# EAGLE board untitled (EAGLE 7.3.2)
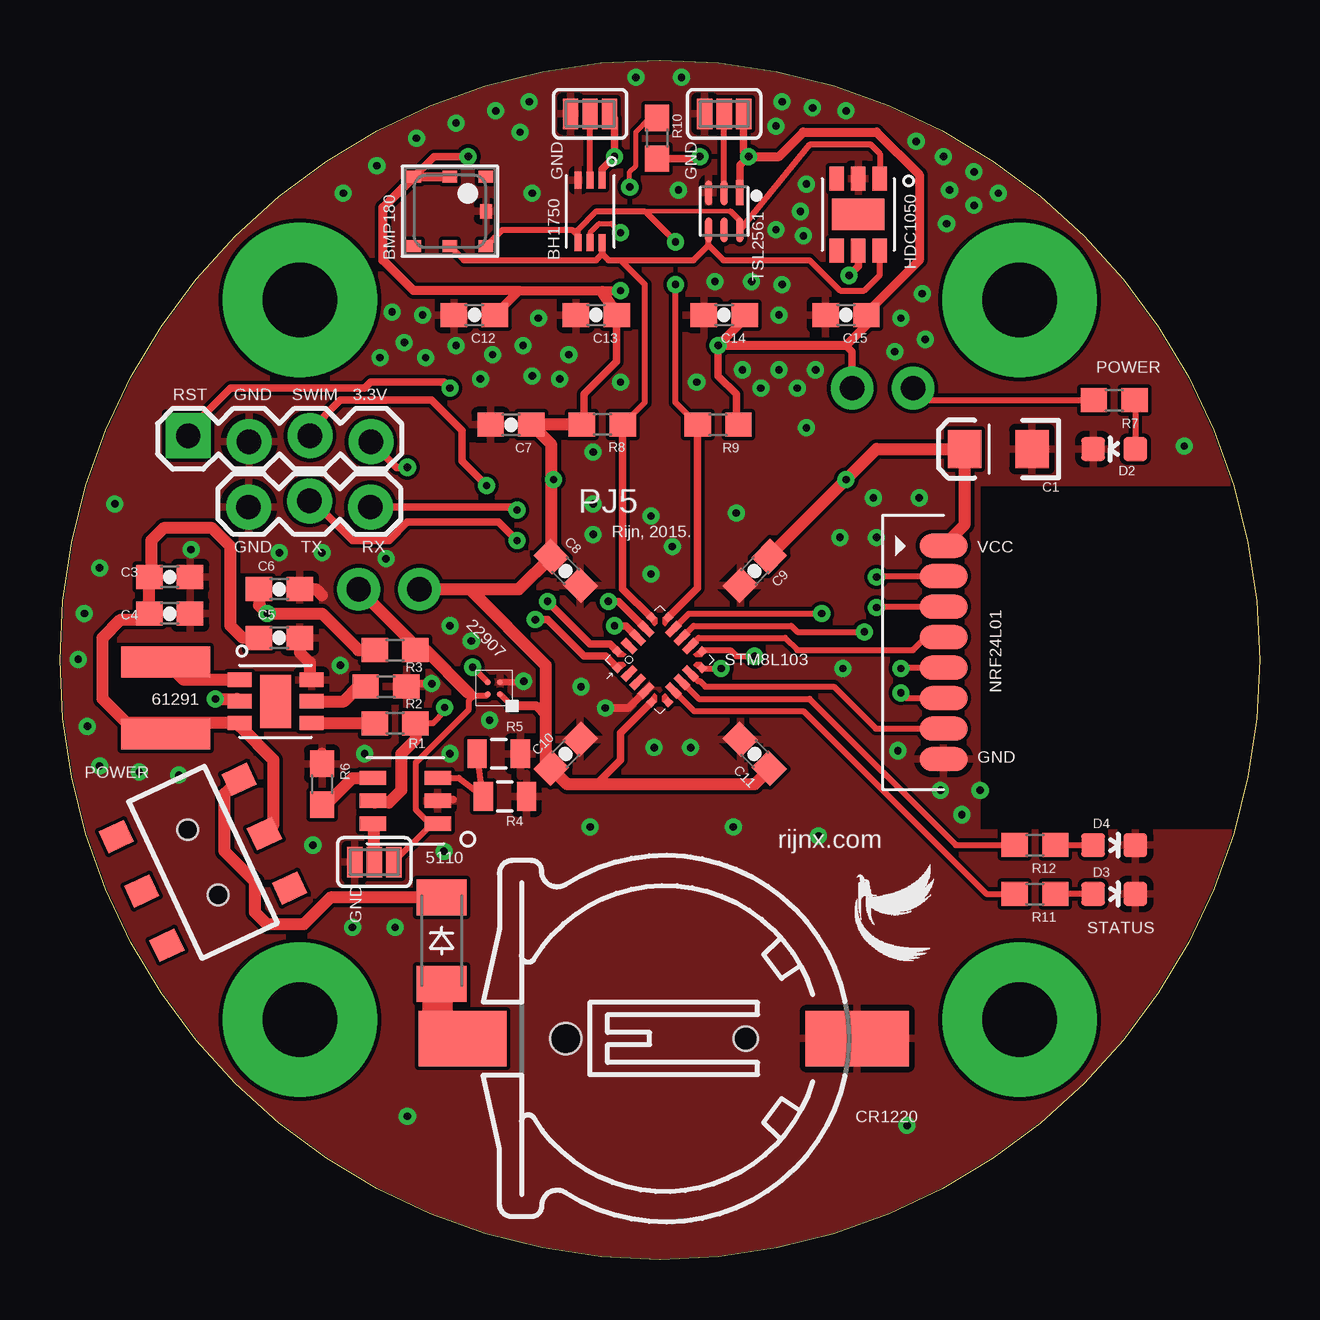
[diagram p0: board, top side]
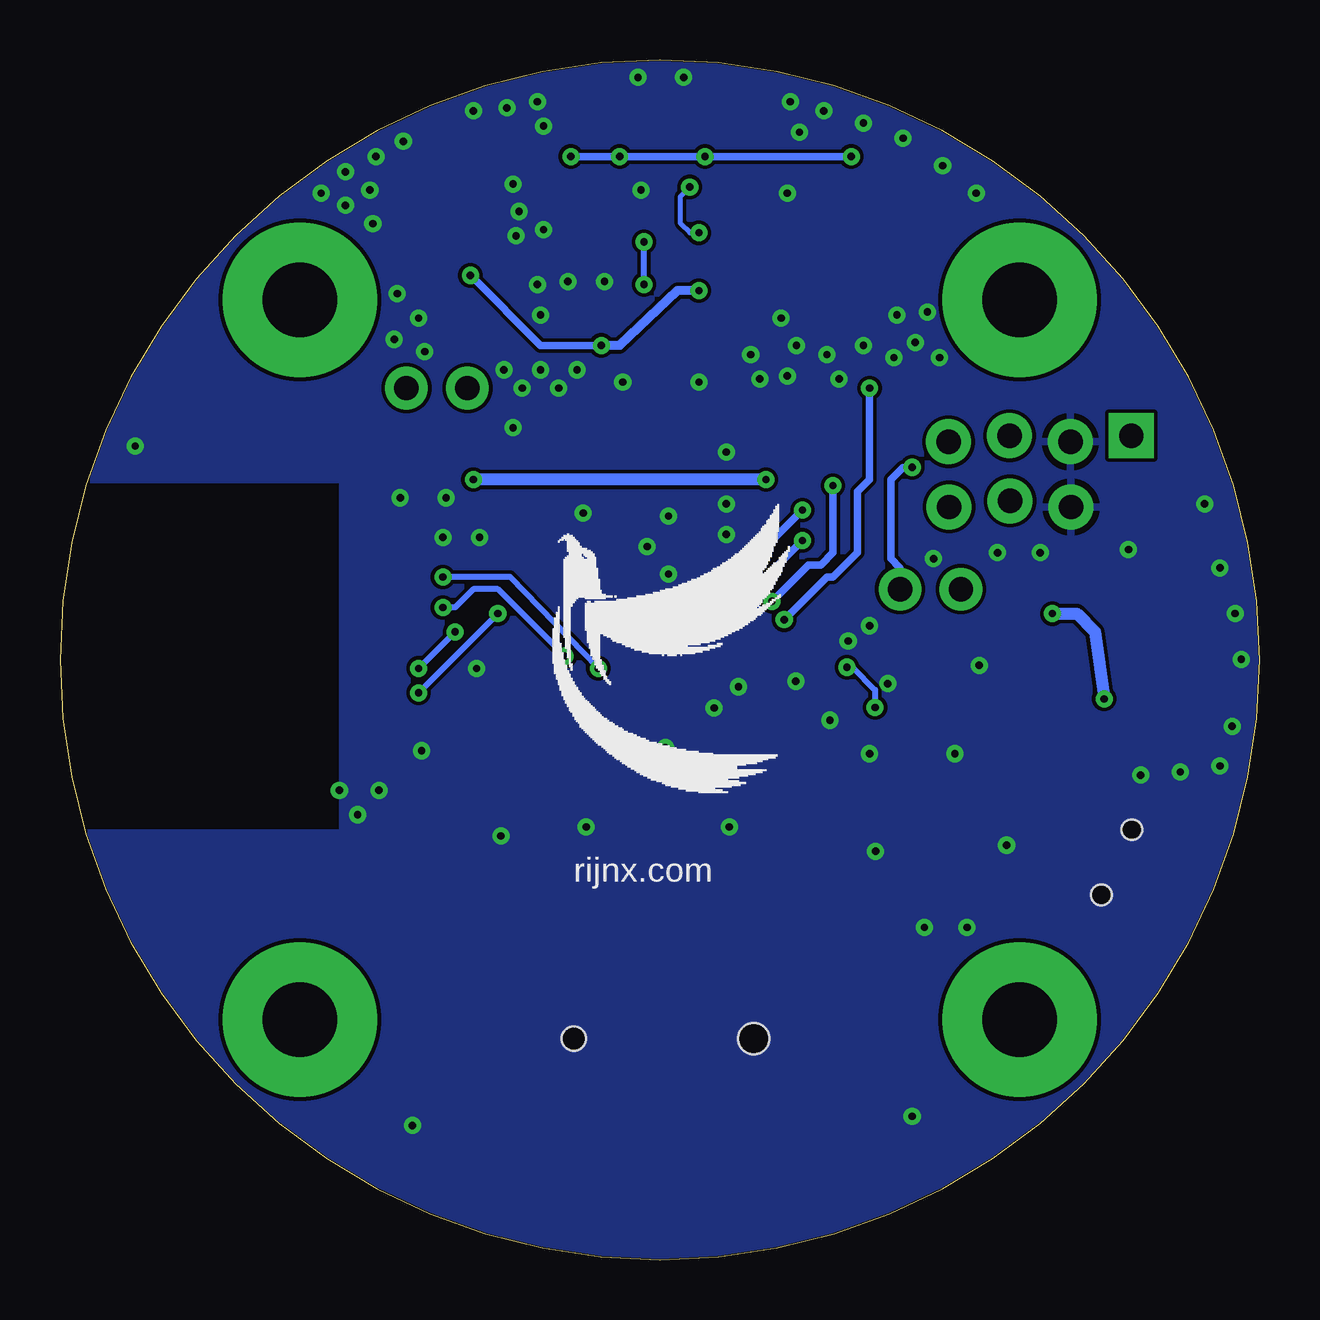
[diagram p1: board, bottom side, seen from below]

Size 50 x 50 mm. Coordinates in mm from the lower left corner, seen from the top.
Outline: 25,50 arc-180 25,0 arc-180 25,50
Copper layers (1*16): Top 0.035mm / dielectric 1.5mm / Bottom 0.035mm
Design rules "default *": minimum track width 6mil, minimum drill 12mil, track to track 6mil, track to pad 6mil, pad to pad 6mil, via to via 6mil, smd to smd 6mil, copper to edge 2mil, drill to drill 6mil, minimum pad ring 10mil, minimum via ring 8mil, stop-mask expansion 4mil, vias tented up to drill 15mil, thermal gap 10mil

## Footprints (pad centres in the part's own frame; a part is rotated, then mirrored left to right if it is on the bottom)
EIA3216 = smd 1.4 x 1.6: A 1.4,0; C -1.4,0
0603-CAP = smd 1.1 x 1: 1 -0.85,0; 2 0.85,0
SOD-123_MINI-SMA = smd 1.5 x 2.1: A 1.8,0; C -1.8,0
LED-0603 = smd 1 x 1: A 0,-0.877; C 0,0.877
CH291-1220LF = smd 2.3 x 3.66: + 0,-2.296 | smd 2.3 x 4.3: - 0,14.146 | hole 1.3: 0,2 | hole 1: 0,9.5
1X03_LOCK = drill 1.016 pad 1.88: 1 0,0.127; 2 2.54,-0.127; 3 5.08,0.127
1X04_LOCK = drill 1.016 pad 1.88 square: 1 0,0.127 | drill 1.016 pad 1.88: 2 2.54,-0.127; 3 5.08,0.127; 4 7.62,-0.127
0603 = smd 1.1 x 1: 1 -0.85,0; 2 0.85,0
0805 = smd 0.8 x 1.2: 1 -0.9,0; 2 0.9,0
AYZ0202 = smd 1 x 1.15: 1 -2.5,2.825; 2 0,2.825; 3 2.5,2.825; 4 -2.5,-2.825; 5 0,-2.825; 6 2.5,-2.825 | hole 0.85: 1.5,0; -1.5,0
PAD-JUMPER-3-NC_BY_PASTE_YES_SILK_FULL_BOX = smd 0.635 x 1.27: 1 -0.813,0; 2 0,0; 3 0.813,0
PTH-JUMPER-2-NO_NO_SILK = drill 1.016 pad 1.778: 1 -1.27,0; 2 1.27,0
BMP180 = smd 0.6 x 0.5: 1 1.5,1.45; 2 0,1.45; 3 -1.5,1.45; 4 -1.5,-1.45; 5 0,-1.45; 6 1.5,-1.45 | smd 0.5 x 0.6: 7 1.5,0
FN-6 = smd 1.05 x 0.3: 1 -0.775,0.65; 2 -0.775,0; 3 -0.775,-0.65; 4 0.775,-0.65; 5 0.775,0; 6 0.775,0.65
SWPA4018S = smd 1.3 x 3.7: P$1 -1.5,0; P$2 1.5,0
PWSON-N6 = smd 0.6 x 1: P$1 0.9,1.5; P$2 0,1.5; P$3 -0.9,1.5; P$4 -0.9,-1.5; P$5 0,-1.5; P$6 0.9,-1.5 | smd 2.2 x 1.3: P$7 0,0
DDC(R-PDSO-G6) = smd 0.6 x 1.1: P$1 -0.95,-1.35; P$2 0,-1.35; P$3 0.95,-1.35; P$4 0.95,1.35; P$5 0,1.35; P$6 -0.95,1.35
YZT(S-XBGA-N4) = smd 0.25 x 0.25: P$A1 0.25,-0.25; P$A2 -0.25,-0.25; P$B1 0.25,0.25; P$B2 -0.25,0.25
UFQFPN20 = smd 0.3 x 0.3: P$1 -1.5,1; P$5 -1.5,-1; P$6 -1,-1.5; P$10 1,-1.5; P$11 1.5,-1; P$15 1.5,1; P$16 1,1.5; P$20 -1,1.5 | smd 0.7 x 0.3: P$2 -1.3,0.5; P$3 -1.3,0; P$4 -1.3,-0.5; P$12 1.3,-0.5; P$13 1.3,0; P$14 1.3,0.5 | smd 0.3 x 0.7: P$7 -0.5,-1.3; P$8 0,-1.3; P$9 0.5,-1.3; P$17 0.5,1.3; P$18 0,1.3; P$19 -0.5,1.3
M08-1.27 = smd 1 x 2: P$1 0,0; P$2 1.27,0; P$3 2.54,0; P$4 3.81,0; P$5 5.08,0; P$6 6.35,0; P$7 7.62,0; P$8 8.89,0
WSOF-6 = smd 0.3 x 0.7: P$1 -0.5,-1.3; P$2 0,-1.3; P$3 0.5,-1.3; P$4 0.5,1.3; P$5 0,1.3; P$6 -0.5,1.3

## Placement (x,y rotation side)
C1  10uF  [EIA3216]  39.12,33.78 180 top
C3  100pF  [0603-CAP]  4.57,28.45 0 top
C4  0.1uF  [0603-CAP]  4.57,26.92 0 top
C5  10uF  [0603-CAP]  9.14,25.91 0 top
C6  22uF  [0603-CAP]  9.14,27.94 0 top
C7  1.0uF  [0603-CAP]  18.8,34.8 180 top
C8  0.1uF  [0603-CAP]  21.08,28.7 315 top
C9  0.1uF  [0603-CAP]  28.96,28.7 225 top
C10  0.1uF  [0603-CAP]  21.08,21.08 45 top
C11  0.1uF  [0603-CAP]  28.96,21.08 135 top
C12  0.1uF  [0603-CAP]  17.27,39.37 180 top
C13  0.1uF  [0603-CAP]  22.35,39.37 180 top
C14  0.1uF  [0603-CAP]  27.69,39.37 180 top
C15  0.1uF  [0603-CAP]  32.77,39.37 180 top
D1  B0520LW  [SOD-123_MINI-SMA]  15.91,13.29 270 top
D2  Yellow  [LED-0603]  43.94,33.78 90 top
D3  Yellow  [LED-0603]  43.94,15.24 270 top
D4  Yellow  [LED-0603]  43.94,17.27 270 top
G1  CH291-1220LF  [CH291-1220LF]  19.08,9.21 270 top
JP1  [1X03_LOCK]  12.94,31.49 180 top
JP2  [1X04_LOCK]  5.34,34.21 0 top
R1  0  [0603]  13.97,22.35 180 top
R2  0  [0603]  13.59,23.88 180 top
R3  0  [0603]  13.97,25.4 180 top
R4  40.2K  [0805]  18.54,19.3 180 top
R5  48.7K  [0805]  18.29,21.08 180 top
R6  10K  [0603]  10.92,19.81 270 top
R7  500  [0603]  43.94,35.81 180 top
R8  4.7K  [0603]  22.61,34.8 0 top
R9  4.7K  [0603]  27.43,34.8 180 top
R10  1K  [0603]  24.89,46.74 270 top
R11  500  [0603]  40.64,15.24 180 top
R12  500  [0603]  40.64,17.27 180 top
S1  AYZ0202  [AYZ0202]  5.96,16.56 295 top
SJ1  JUMPER-PAD-3-NC_BY_PASTE  [PAD-JUMPER-3-NC_BY_PASTE_YES_SILK_FULL_BOX]  13.1,16.57 180 top
SJ2  JUMPER-BYPASS  [PTH-JUMPER-2-NO_NO_SILK]  13.72,27.94 180 top
SJ3  JUMPER-POWERLED  [PTH-JUMPER-2-NO_NO_SILK]  34.29,36.32 180 top
SJ4  JUMPER-PAD-3-NC_BY_PASTE  [PAD-JUMPER-3-NC_BY_PASTE_YES_SILK_FULL_BOX]  27.69,47.75 180 top
SJ5  JUMPER-PAD-3-NC_BY_PASTE  [PAD-JUMPER-3-NC_BY_PASTE_YES_SILK_FULL_BOX]  22.1,47.75 0 top
U1  BMP180  [BMP180]  16.26,43.69 0 top
U2  TSL2561FN  [FN-6]  27.69,43.69 270 top
U$1  SWPA4018S3R3MT  [SWPA4018S]  4.41,23.41 90 top
U$2  TPS61291  [PWSON-N6]  8.98,23.27 90 top
U$3  TPL5110  [DDC(R-PDSO-G6)]  14.4,19.12 90 top
U$4  TPS22907  [YZT(S-XBGA-N4)]  18.09,23.81 0 top
U$5  STM8L101  [UFQFPN20]  25,25 45 top
U$6  NRF24L01_MODULE_SMD  [M08-1.27]  36.83,29.75 270 top
U$7  HDC1050  [PWSON-N6]  33.27,43.56 0 top
U$8  BH1750  [WSOF-6]  22.1,43.69 180 top
U$9  [LOGO-3]  29.51,19.41 0 bottom
U$10  [LOGO-1]  33.12,12.43 0 top

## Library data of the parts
C1 = SparkFun-Capacitors; PROD_ID: CAP-00811
C3-C6 = SparkFun-Capacitors; PROD_ID: CAP-07883
C7 = SparkFun-Capacitors; PROD_ID: CAP-00868
C8-C15 = SparkFun-Capacitors; PROD_ID: CAP-08604
D1 = diode
D2-D4 = SparkFun-LED; PROD_ID: DIO-09003
G1 = battery
JP1 JP2 = SparkFun-Connectors
R1-R3 R6-R12 = SparkFun-Resistors; PROD_ID: RES-08306
R4 R5 = SparkFun-Resistors; PROD_ID: RES-09883
S1 = SparkFun-Electromechanical; PROD_ID: SWCH-08179; SF_ID: COM-00597
SJ1-SJ5 = SparkFun-Passives
U1 U2 = SparkFun-Sensors
U$1-U$4 U$6-U$10 = User-Submitted
U$5 = st-microelectronics; DEVICE: STM8F101

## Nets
3.3V: R3.1 SJ1.1 SJ2.2 U$3.P$1 U$4.P$A2
DONE: R6.2 U$3.P$4
GND: C1.C C3.2 C4.2 C5.2 C6.2 C7.2 C8.2 C9.2 C10.2 C11.2 C12.2 C13.2 C14.2 C15.2 D2.C D3.C D4.C G1.- JP1.3 JP2.2 R2.1 R4.1 R5.1 R6.1 SJ1.3 SJ4.3 SJ5.1 U1.7 U2.3 U$2.P$6 U$3.P$2 U$4.P$B1 U$5.P$4 U$6.P$8 U$7.P$2 U$8.P$3
I2C_INT: U2.5
I2C_SCL: R8.2 U1.5 U2.4 U$5.P$16 U$7.P$6 U$8.P$6
I2C_SDA: R9.2 U1.6 U2.6 U$5.P$15 U$7.P$1 U$8.P$4
MESH: C1.A C7.1 C8.1 C9.1 C10.1 C11.1 C12.1 C13.1 C14.1 C15.1 JP2.4 R8.1 R9.1 R10.2 SJ2.1 SJ3.2 SJ4.1 SJ5.3 U1.2 U1.3 U2.1 U$4.P$A1 U$5.P$5 U$6.P$1 U$7.P$5 U$8.P$1
N$1: D1.A G1.+
N$2: D1.C S1.1
N$3: U$1.P$2 U$2.P$1
N$4: C6.1 R3.2 U$2.P$2
N$5: R1.2 U$2.P$4
N$6: R2.2 U$2.P$5
N$7: R4.2 R5.2 U$3.P$3
N$8: R7.2 SJ3.1
N$9: D2.A R7.1
N$10: SJ1.2 U$3.P$6
N$11: SJ4.2 U2.2
N$12: SJ5.2 U$8.P$2
N$13: R10.1 U$8.P$5
N$14: D3.A R11.1
N$15: D4.A R12.1
N$16: R11.2 U$5.P$7
N$17: R12.2 U$5.P$8
NRF_CE: U$5.P$10 U$6.P$2
NRF_CSN: U$5.P$11 U$6.P$3
NRF_IRQ: U$5.P$9 U$6.P$7
RST: JP2.1 U$5.P$1
SPI_MISO: U$5.P$14 U$6.P$6
SPI_MOSI: U$5.P$13 U$6.P$5
SPI_SCK: U$5.P$12 U$6.P$4
SWIM: JP2.3 U$5.P$20
TPL_DRV: R1.1 U$3.P$5 U$4.P$B2
UART_RX: JP1.1 U$5.P$17
UART_TX: JP1.2 U$5.P$18
V_BATT: C3.1 C4.1 C5.1 S1.2 U$1.P$1 U$2.P$3

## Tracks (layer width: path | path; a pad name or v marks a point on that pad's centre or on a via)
3.3V
  Top 0.254: 17.02,23.62 17.17,23.62 17.27,23.52 | 17.27,23.52 17.8,23.52 U$4.P$A2 | U$3.P$1 15.4,18.17 | 15.4,18.17 14.83,18.75 14.83,20.73 17.04,22.94 17.04,23.29 17.27,23.52 | 15.4,18.17 15.4,18.06 SJ1.1
  Top 0.508: SJ2.2 14.82,25.57 R3.1 15.24,25.4 17.02,23.62
DONE
  Top 0.508: R6.2 11.09,18.96 12.19,20.07 U$3.P$4
GND  (via drill 0.3)
  Top 0.254: U$4.P$B1 19.29,24.06 v19.33,24.11
  Top 0.305: R2.1 14.95,24 v15.49,24 | U$3.P$2 15.8,19.18 16.38,19.18 | U$5.P$4 23.69,22.99 v22.73,22.99
  Top 0.508: C5.2 9.99,25.31 10.41,24.89 10.41,24.24 U$2.P$6 | C6.2 10.67,27.94 10.92,27.69 | R6.1 10.92,21.08
  other vias: 11.68,24.77 21.21,37.72 19.68,36.83 18.03,37.72 14.35,38.23 11.81,44.45 19.68,44.45 30.1,48.26 30.1,40.64 25.78,44.58 16.26,26.42 17.14,25.78 22.23,31.5 22.23,30.23 22.23,33.66 2.29,31.5 5.46,29.59 17.91,22.48 21.72,23.88 24.77,21.34 26.29,21.34 31.62,17.65 14.48,5.97 35.31,5.59 28.19,31.11 24.64,30.99 25.53,29.72 24.64,28.57 22.1,18.03 28.07,18.03 32.51,30.1 32.64,24.64 34.92,21.21 34.04,30.1 33.91,31.75 35.81,31.75 46.86,33.91 36.7,19.56 38.35,19.56 37.59,18.54 1.65,28.83 1.02,26.92 0.76,25.02 1.14,22.23 1.65,20.57 3.3,20.32 4.95,20.19 10.54,17.27 9.14,29.46 10.92,29.46 13.59,29.21 12.19,13.84 13.97,13.84 16,17.02 16.26,21.08 31.11,34.67 13.21,45.59 14.86,46.74 16.51,47.37 18.16,47.88 19.56,48.26 19.18,46.99 24,49.28 25.91,49.28 31.37,48.01 32.77,47.88 29.84,47.24 35.69,46.61 36.83,45.97 38.1,45.34 39.12,44.45 37.08,44.58 38.1,43.94 36.96,43.18 35.94,40.26 35.05,39.24 36.07,38.35 34.8,37.85 13.84,39.5 15.11,39.37 13.34,37.59 15.24,37.59 16.51,38.1 17.53,36.7 19.94,39.24 19.3,38.1 20.83,36.7 23.37,36.58 26.54,36.58 28.45,37.08 29.21,36.32 29.97,37.08 30.73,36.32 31.5,37.08 30.86,43.69 29.84,42.93 30.99,42.67 27.3,40.77 28.83,40.77 29.97,39.37 12.7,21.08 31.11,44.83
  pour Top: -1.27,51.31 50.8,51.31 50.8,32.38 38.23,32.38 38.23,17.78 50.93,17.78 50.93,-0.64 -1.27,-0.64
  pour Bottom: 0.13,53.72 53.09,53.72 53.09,32.51 38.23,32.51 38.23,17.78 50.93,17.78 50.93,-0.51 -0.38,-0.51 -0.38,53.72
I2C_SCL
  Top 0.254: U1.5 16.84,41.66 22.35,41.66 22.6,41.9 U$8.P$6 22.61,41.91 22.86,41.66 23.37,41.66 | 23.37,41.66 26.42,41.66 27.04,42.28 | 27.04,42.28 U2.4 | 27.04,42.28 27.66,41.66 31.24,41.66 32.51,40.39 33.53,40.39 34.17,41.03 U$7.P$6 | R8.2 24.38,35.73 24.38,40.64 23.37,41.66
  Top 0.305: U$5.P$16 23.46,27.96 R8.2
I2C_SDA  (via drill 0.3)
  Top 0.178: 27.94,43.69 23.75,43.69
  Top 0.254: U1.6 18.44,42.93 21.34,42.93 21.59,42.67 | 21.59,42.67 21.6,42.66 U$8.P$4 21.59,42.67 | 21.59,42.67 21.59,42.93 22.35,43.69 23.75,43.69 24.38,43.69 v25.65,42.42 | 27.94,43.69 28.34,43.29 U2.6 31.27,46.48 33.78,46.48 34.17,46.09 U$7.P$1 | R9.2 25.65,35.73 v25.65,40.64
  Top 0.305: U$5.P$15 26.58,28 R9.2
  Bottom 0.254: v25.65,40.64 v25.65,42.42
MESH  (via drill 0.3)
  Top 0.178: v20.57,32.51 20.48,32.6 20.48,33.53
  Top 0.254: U$4.P$A1 18.82,23.09
  Top 0.305: U$8.P$1 22.6,45.46 v23.11,45.97 23.11,47.55 SJ5.3 | v17.02,45.97 15.59,45.97 U1.3 | U2.1 28.34,45.61 v28.7,45.97 28.5,46.18 SJ4.1 | U$7.P$5 33.27,41.4 v32.89,41.02 | R10.2 26.58,45.89 v26.67,45.97 | C13.1 23.2,37.43 21.84,36.07 21.84,34.89 R8.1 | v27.43,38.1 27.43,36.83 28.19,36.07 28.19,34.89 R9.1 | SJ3.2 33.02,37.85 32.77,38.1 | U$5.P$5 23.37,21.95 23.37,20.83 22.35,19.81 | JP2.4 14.03,33.02 v14.48,33.02
  Top 0.381: 18.82,23.09 19.84,23.09 20.24,22.68 | C12.1 19.14,40.39 | 19.14,40.39 22.61,40.39 | 22.61,40.39 23.2,39.54 C13.1 22.61,40.22 22.61,40.39 | 22.61,40.39 v23.37,40.39 | C14.1 28.54,39.2 v27.43,38.1 32.77,38.1 33.62,38.95 C15.1 | 19.14,40.39 14.73,40.39 13.46,41.66 13.46,43.84 U1.3 U1.2 | v28.7,45.97 29.97,45.97 30.99,46.99 34.04,46.99 35.81,45.21 35.81,41.66 33.53,39.37
  Top 0.508: C9.1 v32.77,32.51 34.04,33.78 C1.A 37.72,30.64 U$6.P$1 | R8.1 C7.1 20.48,33.96 20.48,33.53 C8.1 19.12,27.94 SJ2.1 17.07,27.94 20.24,24.77 20.24,22.68 20.24,20.72 C10.1 21.15,19.81 22.35,19.81 28.96,19.81 29.56,20.41 C11.1
  Bottom 0.305: v17.02,45.97 v23.11,45.97 v26.67,45.97 v28.7,45.97 | v32.89,41.02 29.97,38.1 v27.43,38.1 | v14.48,33.02 14.86,33.02 15.37,32.51 15.37,29.21 14.99,28.83 SJ2.1
  Bottom 0.381: v23.37,40.39 24.26,40.39 26.67,38.1 v27.43,38.1
  Bottom 0.508: v20.57,32.51 v32.77,32.51
N$1
  Top 1.27: D1.A 15.75,11.49 15.75,9.65 16.79,9.65 G1.+
N$2
  Top 0.508: D1.C 11.28,15.09 10.16,13.97 8.64,13.97 8.13,14.48 8.13,15.75 6.86,17.02 6.86,19.41 S1.1
N$3
  Top 0.508: U$2.P$1 5.16,24.17 U$1.P$2
N$4  (via drill 0.3)
  Top 0.508: C6.1 8.29,27.27 v8.64,26.92 10.92,26.92 12.45,25.4 R3.2 | v6.48,23.37 7.38,23.37 U$2.P$2
  Bottom 0.508: v8.64,26.92 7.62,26.92 6.86,26.16 v6.48,23.37
N$5
  Top 0.508: U$2.P$4 13.11,22.37 R1.2
N$6
  Top 0.508: U$2.P$5 11.84,23.27 12.45,23.88 R2.2
N$7
  Top 0.254: U$3.P$3 16.62,20.07 R4.2 R5.2
N$8
  Top 0.254: SJ3.1 36.07,35.81 R7.2
N$9
  Top 0.254: R7.1 44.82,35.79 D2.A
N$10
  Top 0.508: SJ1.2 13.1,18.12 U$3.P$6
N$11
  Top 0.254: U2.2 SJ4.2
N$12
  Top 0.254: U$8.P$2 SJ5.2
N$13  (via drill 0.3)
  Top 0.203: U$8.P$5 22.1,42.8 22.48,43.18 22.99,43.18 v23.37,42.8 | v23.75,44.7 23.75,45.34 24,45.59 24,46.99 24.6,47.59 R10.1
  Bottom 0.203: v23.37,42.8 23.75,42.8 24.13,43.18 24.13,44.32 v23.75,44.7
N$14
  Top 0.254: D3.A R11.1
N$15
  Top 0.254: R12.1 D4.A
N$16
  Top 0.254: U$5.P$7 26.43,22.86 30.99,22.86 38.61,15.24 R11.2
N$17
  Top 0.254: U$5.P$8 26.63,23.37 31.24,23.37 37.34,17.27 R12.2
N$18  (via drill 3.1 pad 6.45)
  other vias: 40,40
N$19  (via drill 3.1 pad 6.45)
  other vias: 40,10
N$20  (via drill 3.1 pad 6.45)
  other vias: 10,10
N$21  (via drill 3.1 pad 6.45)
  other vias: 10,40
NRF_CE  (via drill 0.3)
  Top 0.254: U$5.P$10 26.78,24.64 v27.56,24.64 | v34.04,28.45 34.07,28.48 U$6.P$2
  Bottom 0.254: v27.56,24.64 31.24,28.45 v34.04,28.45
NRF_CSN  (via drill 0.3)
  Top 0.254: U$5.P$11 26.81,25.4 27.94,25.4 28.19,25.15 v28.96,25.15 | v34.04,27.18 34.07,27.21 U$6.P$3
  Bottom 0.254: v28.96,25.15 31.75,27.94 32.77,27.94 33.53,27.18 v34.04,27.18
NRF_IRQ
  Top 0.254: U$5.P$9 26.6,24.11 26.67,24.11 26.9,23.88 32.26,23.88 34,22.13 U$6.P$7
RST  (via drill 0.3)
  Top 0.305: U$5.P$1 22.73,25.15 21.84,25.15 20.32,26.67 v19.81,26.67 | v16.26,36.32 16,36.58 12.95,36.58 12.7,36.32 7.11,36.32 5.34,34.55 JP2.1
  Bottom 0.305: v19.81,26.67 18.03,28.45 17.78,28.45 16.76,29.46 16.76,32 16.26,32.51 v16.26,36.32
SPI_MISO  (via drill 0.3)
  Top 0.254: U$5.P$14 26.22,26.92 v31.75,26.92 | v35.05,23.62 35.27,23.4 U$6.P$6
  Bottom 0.254: v31.75,26.92 v35.05,23.62
SPI_MOSI  (via drill 0.3)
  Top 0.254: U$5.P$13 26.42,26.42 30.48,26.42 30.73,26.16 v33.53,26.16 | v35.05,24.64 35.08,24.67 U$6.P$5
  Bottom 0.254: v33.53,26.16 v35.05,24.64
SPI_SCK
  Top 0.254: U$5.P$12 26.61,25.91 30.23,25.91 30.73,25.4 35.56,25.4 36.1,25.94 U$6.P$4
SWIM  (via drill 0.3)
  Top 0.305: U$5.P$20 22.93,25.65 22.1,25.65 v20.32,27.43 | v17.78,32.26 16.76,33.27 16.76,34.54 15.49,35.81 11.68,35.81 10.42,34.55 JP2.3
  Bottom 0.305: v20.32,27.43 18.8,28.96 18.29,28.96 17.78,29.46 v17.78,32.26
TPL_DRV  (via drill 0.3)
  Top 0.254: U$4.P$B2 17.82,24.06 v17.2,24.69 | v16.03,23.01 16.03,22.84 15.54,22.35 R1.1
  Top 0.508: R1.1 14.82,21.68 14.22,21.08 14.22,19.56 13.72,19.05 13.12,19.05 U$3.P$5
  Bottom 0.254: v17.2,24.69 16.97,24.69 16.03,23.75 v16.03,23.01
UART_RX  (via drill 0.3)
  Top 0.305: U$5.P$17 23.27,27.43 v22.86,27.43 | v19.05,31.24 18.93,31.37 JP1.1
  Bottom 0.305: v22.86,27.43 v19.05,31.24
UART_TX  (via drill 0.3)
  Top 0.305: U$5.P$18 23.58,26.42 v23.11,26.42 | v19.05,29.97 18.29,30.73 14.48,30.73 13.72,29.97 12.19,29.97 10.54,31.62 JP1.2
  Bottom 0.305: v23.11,26.42 22.61,26.42 v19.05,29.97
V_BATT
  Top 0.508: U$2.P$3 4.87,22.37 U$1.P$1 | U$2.P$3 7.48,22.23 8.89,20.83 8.89,18.12 S1.2 | U$2.P$3 2.78,22.37 1.78,23.37 1.78,25.91 2.54,26.67 3.47,26.67 C4.1 C3.1 3.81,28.54 3.81,29.97 4.32,30.48 6.35,30.48 7.11,29.72 7.11,26.42 7.62,25.91 C5.1

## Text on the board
tNames: GND | GND | BMP180 | BH1750 | TSL2561 | HDC1050 | POWER | RST | GND | SWIM | 3.3V | PJ5 | Rijn, 2015. | GND | TX | RX | VCC | 22907 | STM8L103 | NRF24L01 | 61291 | GND | POWER | 5110 | rijnx.com | GND | STATUS | CR1220
bNames: rijnx.com

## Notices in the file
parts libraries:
SparkFun-Capacitors: Licensing: Creative Commons ShareAlike 4.0 International - https://creativecommons.org/licenses/by-sa/4.0
